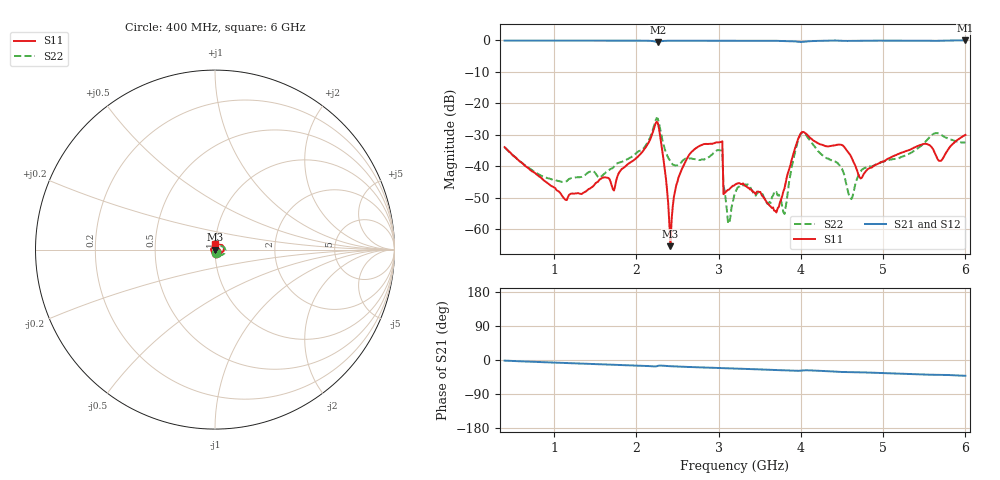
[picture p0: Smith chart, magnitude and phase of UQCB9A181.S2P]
!  Part Number  UQCB9A181	Mounting Orientation: Vertical
!  Description: RF capacitors
!  Application: Coupling, Bypass, Tuning, DC Block
!  Filters, Matching
# GHZ S DB R 50
! Freq  |S11|  S11 Ph  |S21|  S21 Ph  |S12|  S12 Ph  |S22|  S22 Ph
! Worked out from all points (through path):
!   401 points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, 400 MHz to 6 GHz, reference 50 ohm
!   highest |S21| = -0.01 dB at 6 GHz (marker M1); lowest = -0.5 dB at 2.262 GHz (marker M2)
!   group delay of S21, straight-line fit = 19.3 ps
!   lowest |S11| = -65.3 dB at 2.416 GHz (marker M3), VSWR 1.00, Z = 49.9 - j0.00321 ohm
!   |S11| at or under -10 dB: start of sweep to end of sweep
!   |S22| runs from -58.1 to -24.6 dB; largest |S21 - S12| = 0.0023
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0.4  -33.89 -78.5  -0.05 -1.6  -0.04 -1.6  -33.94 -78.3
1.338  -48.76 29.5  -0.06 -9.3  -0.06 -9.3  -43.33 9.5
1.73  -47.64 70.3  -0.08 -12.3  -0.08 -12.3  -40.06 37.0
2.262  -26.26 -8.4  -0.52 -15.5  -0.51 -15.5  -24.85 -21.8
2.276  -27.94 -28.0  -0.42 -14.8  -0.42 -14.8  -26.17 -37.6
2.416  -65.32 -176.6  -0.09 -16.4  -0.09 -16.4  -38.45 -38.0
2.542  -41.64 112.5  -0.08 -17.6  -0.07 -17.6  -38.87 -5.4
2.766  -33.52 86.7  -0.08 -19.5  -0.08 -19.4  -37.98 -0.5
3.018  -32.31 76.3  -0.13 -21.3  -0.12 -21.3  -34.88 15.3
3.088  -48.15 -27.5  -0.11 -21.7  -0.10 -21.7  -50.73 -36.9
3.116  -47.44 -29.2  -0.11 -22.0  -0.10 -21.9  -58.08 -11.5
3.2  -45.81 -38.5  -0.11 -22.6  -0.10 -22.6  -48.37 46.3
3.704  -54.61 162.2  -0.13 -26.5  -0.13 -26.5  -48.12 -40.8
3.802  -46.94 84.9  -0.17 -27.4  -0.16 -27.4  -55.12 -8.1
3.984  -30.24 -16.4  -0.47 -28.3  -0.46 -28.3  -30.54 -30.9
4.138  -31.45 -108.9  -0.21 -27.7  -0.20 -27.7  -32.69 -115.2
4.474  -33.09 177.4  -0.09 -31.4  -0.08 -31.4  -39.73 -143.5
4.6  -36.36 139.0  -0.16 -31.7  -0.15 -31.7  -49.99 -116.5
4.726  -43.81 147.4  -0.12 -32.5  -0.11 -32.5  -41.76 -66.8
5.076  -37.38 146.0  -0.06 -35.1  -0.06 -35.1  -37.90 -63.0
5.692  -38.28 89.6  -0.10 -39.0  -0.10 -39.0  -29.74 -61.9
6  -30.00 94.9  -0.01 -41.7  -0.01 -41.7  -32.46 -54.4
